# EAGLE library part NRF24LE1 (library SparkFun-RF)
Nordic nRF24LE1 Ultra-low Power Wireless System on Chip The Nordic Semiconductor nRF24LE1 is a 2.4GHz ISM band radio with emhanced 8051 MCU, up to 2Mbps on air data rate, 1.9 to 3.6V supply range, 16-32-bit multiplication-division co-processor (MDU), 16 kBytes of on-chip Flash, 1 kBytes on SRAM, 1 kBytes NV data memory, 512 Bytes NV data memory (extended endurance), Interrupt controller with 18 sources and 4 priority levels, 1 Analog comparator, 10 Bit ADC, Hardware SPI slave and master, UART, three 16-bit timers/counters, AES encryption/decryption co-processor, Random number generator, 2-Wire interface, 2 Channel PWM, 7, 15, or 31 GPIO lines, On-chip hardware debug support for a JTAG debugger.
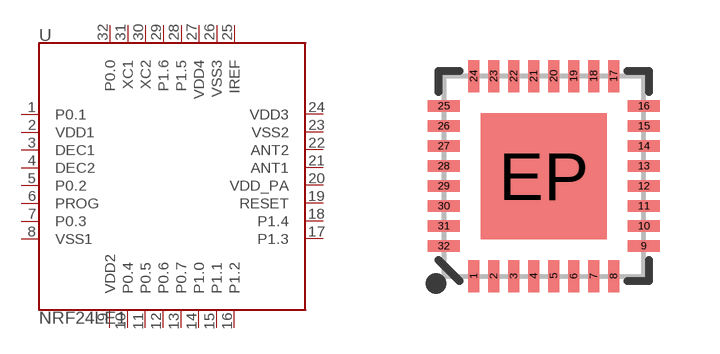
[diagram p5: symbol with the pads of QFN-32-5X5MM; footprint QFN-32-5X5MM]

Designator prefix -

## NRF24LE1 (PROD_ID: IC-09044)  [QFN-32-5X5MM]
1  P0.1
2  VDD1
3  DEC1
4  DEC2
5  P0.2
6  PROG
7  P0.3
8  VSS1
9  VDD2
10  P0.4
11  P0.5
12  P0.6
13  P0.7
14  P1.0
15  P1.1
16  P1.2
17  P1.3
18  P1.4
19  RESET
20  VDD_PA
21  ANT1
22  ANT2
23  VSS2
24  VDD3
25  IREF
26  VSS3
27  VDD4
28  P1.5
29  P1.6
30  XC2
31  XC1
32  P0.0

## Footprint QFN-32-5X5MM (pad centres in mm)
QFN 32-Pin w/ Thermal Pad - 5.0 x 5.0 mm Used by nRF24LU1 and nRF24LE1 Datasheet Example
smd 0.285 x 0.8: 1 -1.75,-2.5; 2 -1.25,-2.5; 3 -0.75,-2.5; 4 -0.25,-2.5; 5 0.25,-2.5; 6 0.75,-2.5; 7 1.25,-2.5; 8 1.75,-2.5; 17 1.75,2.5; 18 1.25,2.5; 19 0.75,2.5; 20 0.25,2.5; 21 -0.25,2.5; 22 -0.75,2.5; 23 -1.25,2.5; 24 -1.75,2.5
smd 0.8 x 0.285: 9 2.5,-1.75; 10 2.5,-1.25; 11 2.5,-0.75; 12 2.5,-0.25; 13 2.5,0.25; 14 2.5,0.75; 15 2.5,1.25; 16 2.5,1.75; 25 -2.5,1.75; 26 -2.5,1.25; 27 -2.5,0.75; 28 -2.5,0.25; 29 -2.5,-0.25; 30 -2.5,-0.75; 31 -2.5,-1.25; 32 -2.5,-1.75
smd 3.15 x 3.15: EP 0,0

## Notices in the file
Licensing: Creative Commons ShareAlike 4.0 International - https://creativecommons.org/licenses/by-sa/4.0
© 2015 RF Digital Corporation
